FUNCTION FC1
TITLE =Read SDO
//*****************************************************************************
//* maxon motor ag
//* R&D
//* all rights reserved
//*****************************************************************************
//* Summary:  Read an object via SDO
//*
//* Remarks:
//*
//* Created under: STEP7 REV5.2+SP1
//*****************************************************************************
//* History:
//* 18.05.2004 | INA   first release
//*
//*
//*****************************************************************************

AUTHOR:INA
FAMILY:SDO
NAME:ReadSDO
VERSION:00.01


VAR_INPUT

NodeID : BYTE //Adress of the maxon device

  Index : DWORD //Index of the object

  SubIndex : DWORD //Subindex of the object

END_VAR
VAR_OUTPUT
  RET_VAL : BOOL //Done

  Err : BOOL //True = Error detected

  ErrNo : DINT //Error number (CAN or/and VIPA!)

END_VAR
VAR_TEMP
  xBusy : BOOL //The read job is not yet completed

  xCanOpenError : DWORD //Return value from SDO transfer

  xRetValue : WORD //VIPA Error

END_VAR

BEGIN

NETWORK
TITLE =
//

// SDO Read
       R    #RET_VAL                     // Done
       R    #Err
       L    0
       T    #ErrNo

sfc   :NOP  0
       CALL SFC219
         Request:=TRUE
         Slot_Master:=B#16#00
         NodeID:=#NodeID
         Transfertyp:=B#16#60            // Read
         Index:=#Index
         Subindex:=#SubIndex
         CanOpenError:=#xCanOpenError
         RetVal:=#xRetValue
         Busy:=#xBusy
         DataBuffer:=P#DB219.DBX 10.0 DWORD 1

       L    1
       U    #xBusy
       SPB  sfc

       S    #RET_VAL                     // Done

       L    W#16#F021
       L    #xRetValue
       <I
       SPBN ok                           // jump if RetValue lower than 0xF021
       L    W#16#F028
       L    #xRetValue
       >I
       SPB  errV                         // jump if xRetValue between 0xF021 and 0xF028

       L    0
       L    #xCanOpenError
       <>D
       SPB  errC                         // jump if CAN error

ok    :NOP  0
       R    #Err
       SPA  end

errC  :NOP  0                            // CANopen error
       S    #Err
       L    #xCanOpenError
       TAD
       T    #ErrNo
       SPA  end

errV  :NOP  0                            // VIPA error
       S    #Err

       L    0
       L    #xCanOpenError
       <>D
       SPBN er

       T    #ErrNo
       SPA  end

er    :L    #xRetValue                   // RetVal
       T    #ErrNo

end   :NOP  0
//      R     A      0.4
END_FUNCTION
